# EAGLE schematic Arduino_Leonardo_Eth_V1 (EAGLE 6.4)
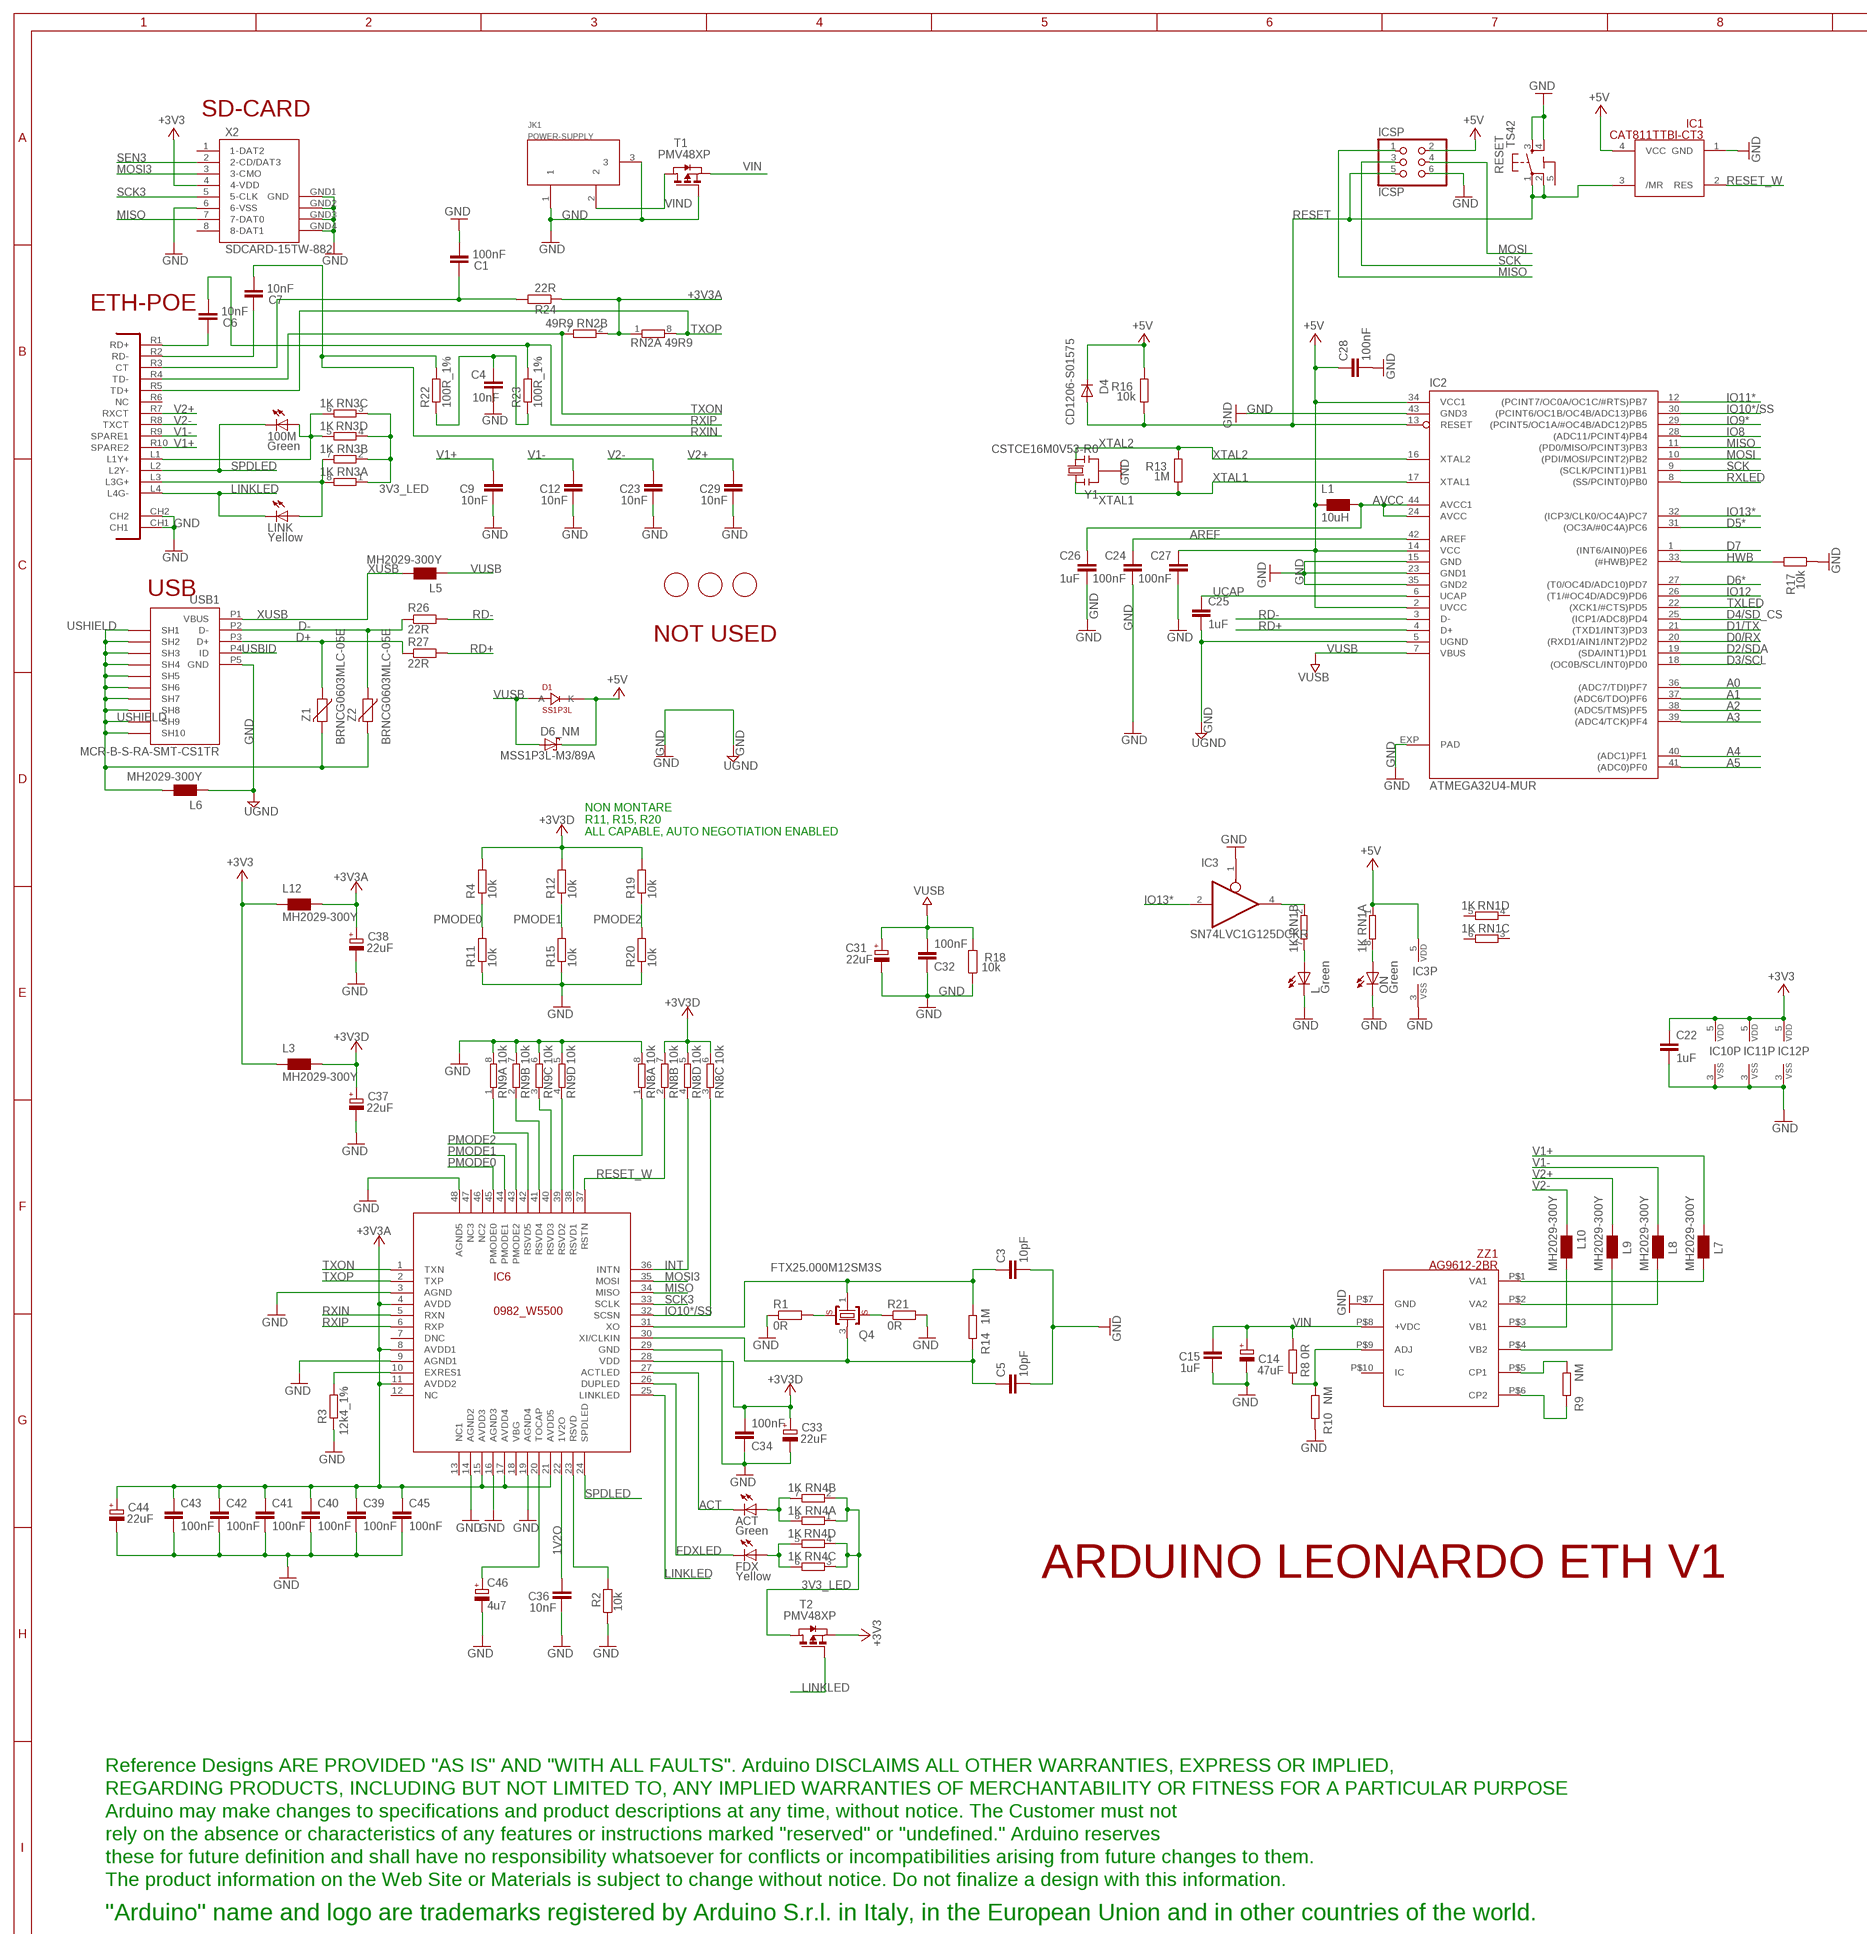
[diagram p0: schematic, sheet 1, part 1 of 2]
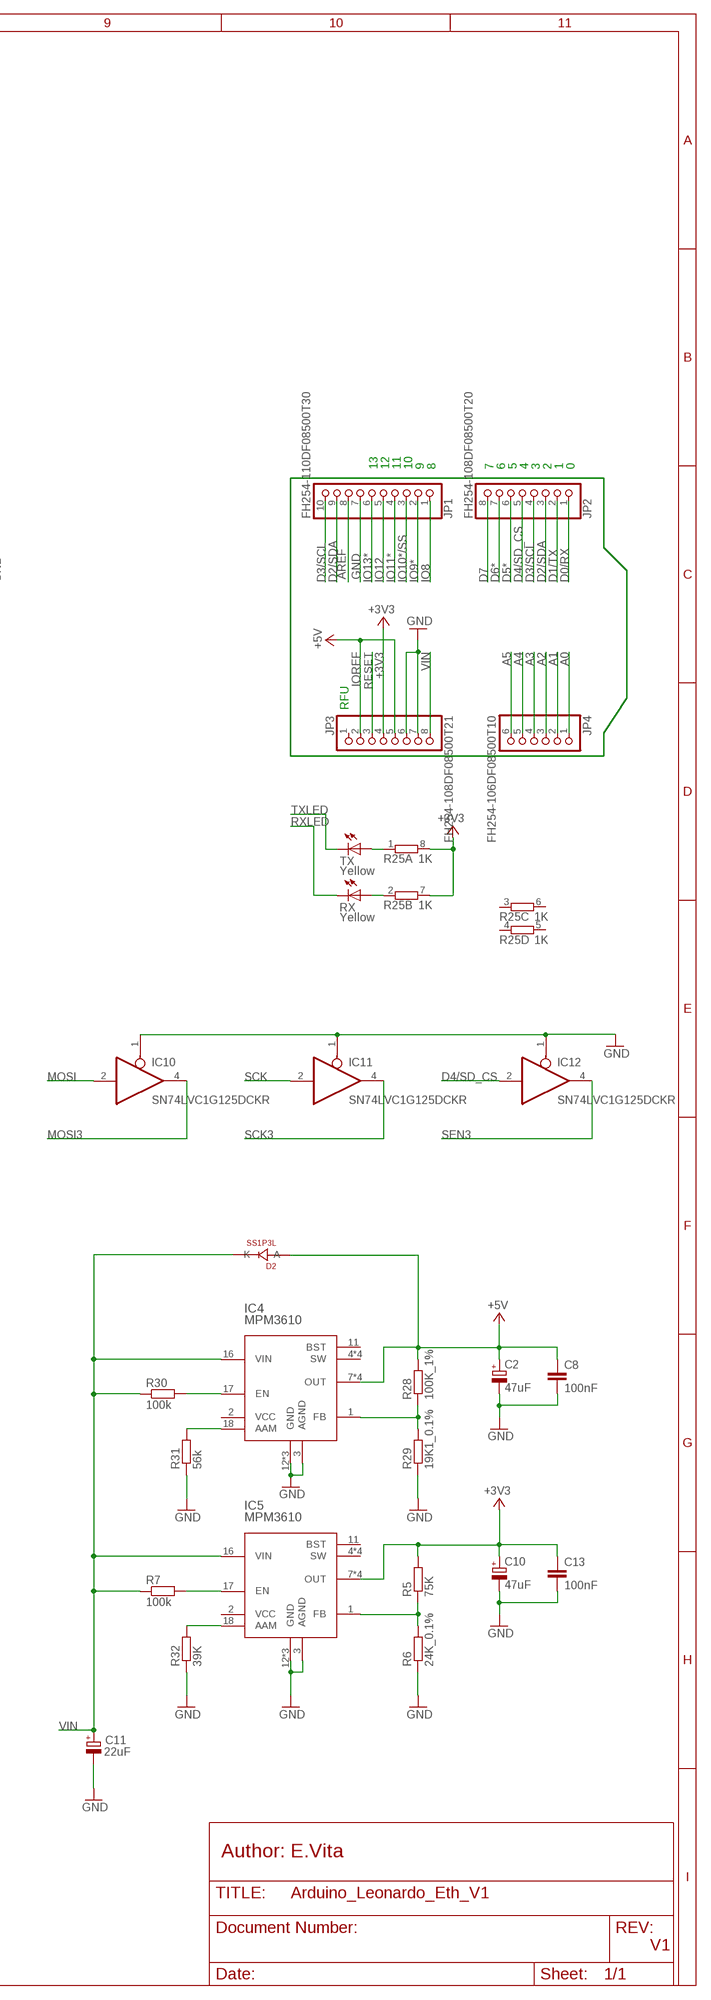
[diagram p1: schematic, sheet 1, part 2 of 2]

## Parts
100M  Green  0043_KPT-2012SGC  [CHIPLED_0805]
ACT  Green  0043_KPT-2012SGC  [CHIPLED_0805]
C1  100nF  0015_100NF_0603  [C0603-ROUND]
C2  47uF  0113_47UF  [PANASONIC_D]
C3  10pF  0245_0603C0G10PF50V  [C0603-ROUND]
C4  10nF  0142_10NF_0603  [C0603-ROUND]
C5  10pF  0245_0603C0G10PF50V  [C0603-ROUND]
C6  10nF  0142_10NF_0603  [C0603-ROUND]
C7  10nF  0142_10NF_0603  [C0603-ROUND]
C8  100nF  0015_100NF_0603  [C0603-ROUND]
C9  10nF  0461_10NF_0805  [C0805K]
C10  47uF  0113_47UF  [PANASONIC_D]
C11  22uF  0167_  [SMC_B]
C12  10nF  0461_10NF_0805  [C0805K]
C13  100nF  0015_100NF_0603  [C0603-ROUND]
C14  47uF  0113_47UF  [PANASONIC_D]
C15  1uF  0006_1UF_0603/GRM188R61E105KA12D  [C0603-ROUND]
C22  1uF  0006_1UF_0603/GRM188R61E105KA12D  [C0603-ROUND]
C23  10nF  0461_10NF_0805  [C0805K]
C24  100nF  0015_100NF_0603  [C0603-ROUND]
C25  1uF  0006_1UF_0603/GRM188R61E105KA12D  [C0603-ROUND]
C26  1uF  0006_1UF_0603/GRM188R61E105KA12D  [C0603-ROUND]
C27  100nF  0015_100NF_0603  [C0603-ROUND]
C28  100nF  0015_100NF_0603  [C0603-ROUND]
C29  10nF  0461_10NF_0805  [C0805K]
C31  22uF  0167_  [SMC_B]
C32  100nF  0015_100NF_0603  [C0603-ROUND]
C33  22uF  0167_  [SMC_B]
C34  100nF  0015_100NF_0603  [C0603-ROUND]
C36  10nF  0142_10NF_0603  [C0603-ROUND]
C37  22uF  0167_  [SMC_B]
C38  22uF  0167_  [SMC_B]
C39  100nF  0015_100NF_0603  [C0603-ROUND]
C40  100nF  0015_100NF_0603  [C0603-ROUND]
C41  100nF  0015_100NF_0603  [C0603-ROUND]
C42  100nF  0015_100NF_0603  [C0603-ROUND]
C43  100nF  0015_100NF_0603  [C0603-ROUND]
C44  22uF  0167_  [SMC_B]
C45  100nF  0015_100NF_0603  [C0603-ROUND]
C46  4u7  0474_TAJA475M016RNJ  [SMC_A]
D1  SS1P3L  0025_SS1P3L-M3/84A  [DO220AAL]
D2  SS1P3L  0025_SS1P3L-M3/84A  [DO220AAL]
D4  CD1206-S01575  0012_CD1206-S01575  [MINIMELF]
D6_NM  MSS1P3L-M3/89A  1653_MSS1P3L-M3/89A  [MICROSMP]
FDX  Yellow  0044_KPT-2012YC  [CHIPLED_0805]
IC1  CAT811TTBI-CT3  0035_CAT811TTBI-GT3  [SOT143]
IC2  ATMEGA32U4-MUR  0159_ATMEGA32U4-MUR  [QFN44ML7X7]
IC3  SN74LVC1G125DCKR  0040_SN74LVC1G125DCKR  [SC70-5]
IC4  MPM3610  2093_MPM3610GQV-P  [QFN-20]
IC5  MPM3610  2093_MPM3610GQV-P  [QFN-20]
IC6  0982_W5500  [TQFP48-7X7]
IC10  SN74LVC1G125DCKR  0040_SN74LVC1G125DCKR  [SC70-5]
IC11  SN74LVC1G125DCKR  0040_SN74LVC1G125DCKR  [SC70-5]
IC12  SN74LVC1G125DCKR  0040_SN74LVC1G125DCKR  [SC70-5]
ICSP  ICSP  0114_PH254-203DF118A00V  [2X03]
JK1  POWER-SUPPLY  0018_19746-POWER-SUPPLY  [POWERSUPPLY_DC-21MM]
JP1  FH254-110DF08500T30  1216_FH254-110DF08500T30  [1X10]
JP2  FH254-108DF08500T20  1218_FH254-108DF08500T20  [1X08]
JP3  FH254-108DF08500T21  1217_FH254-108DF08500T21  [1X08]
JP4  FH254-106DF08500T10  1215_FH254-106DF08500T10_STD  [1X06]
L  Green  0043_KPT-2012SGC  [CHIPLED_0805]
L1  10uH  0715_CV201210-100K  [0805]
L3  MH2029-300Y  0001_BLM21PG300SN1D_/_MH2029-300Y  [0805]
L5  MH2029-300Y  0001_BLM21PG300SN1D_/_MH2029-300Y  [0805]
L6  MH2029-300Y  0001_BLM21PG300SN1D_/_MH2029-300Y  [0805]
L7  MH2029-300Y  0001_BLM21PG300SN1D_/_MH2029-300Y  [0805]
L8  MH2029-300Y  0001_BLM21PG300SN1D_/_MH2029-300Y  [0805]
L9  MH2029-300Y  0001_BLM21PG300SN1D_/_MH2029-300Y  [0805]
L10  MH2029-300Y  0001_BLM21PG300SN1D_/_MH2029-300Y  [0805]
L12  MH2029-300Y  0001_BLM21PG300SN1D_/_MH2029-300Y  [0805]
LINK  Yellow  0044_KPT-2012YC  [CHIPLED_0805]
ON  Green  0043_KPT-2012SGC  [CHIPLED_0805]
Q4  FTX25.000M12SM3S  0846_FTX25.000M12SM3S  [CRYSTAL3.2X2.5]
R1  0R  0039_JUMP_0402  [R0402]
R2  10k  0028_CR0603JW103L  [R0603-ROUND]
R3  12k4_1%  0984_12K4_1%_0603  [R0603-ROUND]
R4  10k  0028_CR0603JW103L  [R0603-ROUND]
R5  75K  0376_CR0603FX7502_L  [R0603-ROUND]
R6  24K_0.1%  2338_  [R0603-ROUND]
R7  100k  0026_100K_0603  [R0603-ROUND]
R8  0R  0233_0R_0603  [R0603-ROUND]
R9  NM  0233_0R_0603  [R0603-ROUND]
R10  NM  0233_0R_0603  [R0603-ROUND]
R11  10k  0028_CR0603JW103L  [R0603-ROUND]
R12  10k  0028_CR0603JW103L  [R0603-ROUND]
R13  1M  0004_0603_1M  [R0603-ROUND]
R14  1M  0004_0603_1M  [R0603-ROUND]
R15  10k  0028_CR0603JW103L  [R0603-ROUND]
R16  10k  0028_CR0603JW103L  [R0603-ROUND]
R17  10k  0028_CR0603JW103L  [R0603-ROUND]
R18  10k  0028_CR0603JW103L  [R0603-ROUND]
R19  10k  0028_CR0603JW103L  [R0603-ROUND]
R20  10k  0028_CR0603JW103L  [R0603-ROUND]
R21  0R  0039_JUMP_0402  [R0402]
R22  100R_1%  0131_CR0603FX1000L  [R0603-ROUND]
R23  100R_1%  0131_CR0603FX1000L  [R0603-ROUND]
R24  22R  0247_22R_0603  [R0603-ROUND]
R25  1K  0005_064R_1K_/_CAY16-102J4LF  [CAY16]
R26  22R  0247_22R_0603  [R0603-ROUND]
R27  22R  0247_22R_0603  [R0603-ROUND]
R28  100K_1%  2022_CR0603FW104L  [R0603-ROUND]
R29  19K1_0.1%  2339_  [R0603-ROUND]
R30  100k  0026_100K_0603  [R0603-ROUND]
R31  56k  0411_56K_0603  [R0603-ROUND]
R32  39K  0756_  [R0603-ROUND]
RESET  TS42  0946_TS42031-160W-TR-7260  [TS42]
RN1  1K  0005_064R_1K_/_CAY16-102J4LF  [CAY16]
RN2  49R9  0036_CAY16-49R9F4L  [CAY16]
RN3  1K  0005_064R_1K_/_CAY16-102J4LF  [CAY16]
RN4  1K  0005_064R_1K_/_CAY16-102J4LF  [CAY16]
RN8  10k  0016_064R_10K_/_CAY16-103J4LF  [CAY16]
RN9  10k  0016_064R_10K_/_CAY16-103J4LF  [CAY16]
RX  Yellow  0044_KPT-2012YC  [CHIPLED_0805]
T1  PMV48XP  0297_PMV48XP  [SOT-23]
T2  PMV48XP  0297_PMV48XP  [SOT-23]
TX  Yellow  0044_KPT-2012YC  [CHIPLED_0805]
U$1  DISCLAIMER  [DISCLAIMER]
U$2  FIDUCIALMOUNT  [FIDUCIA-MOUNT]
U$4  FIDUCIALMOUNT  [FIDUCIA-MOUNT]
U$5  FIDUCIALMOUNT  [FIDUCIA-MOUNT]
UC1  RB1-125BHQ1A  0033_RB1-125BHQ1A  [POE-RJ45]
USB1  MCR-B-S-RA-SMT-CS1TR  0158_MCR-B-S-RA-SMT-CS1TR  [CON2_USB_MICRO_B_AT]
X2  SDCARD-15TW-882  0046_15TW-882  [SDCARD-15TW-8821]
Y1  CSTCE16M0V53-R0  0011_CSTCE16M0V53-R0  [RESONATOR]
Z1  BRNCG0603MLC-05E  0010_BRNCG0603MLC-05E  [CT/CN0603]
Z2  BRNCG0603MLC-05E  0010_BRNCG0603MLC-05E  [CT/CN0603]
ZZ1  AG9612-2BR  0343_AG9612-2BR  [AG9000]

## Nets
1V2O: C36.2 IC6.22(1V2O)
3V3_LED [power]: RN3.1 RN3.2 RN3.3 RN3.4 RN4.1 RN4.2 RN4.3 RN4.4 T2.1(D)
+3V3 [power]: C10.+ C13.1 C22.1 IC5.7(OUT) IC5.8(OUT) IC5.9(OUT) IC5.20(OUT) IC10.5(VDD) IC11.5(VDD) IC12.5(VDD) JP3.4 L3.1 L12.1 R5.2 R25.7 R25.8 T2.2(S) X2.4(4-VDD)
+3V3A [power]: C38.+ C39.1 C40.1 C41.1 C42.1 C43.1 C44.+ C45.1 IC6.4(AVDD) IC6.8(AVDD1) IC6.11(AVDD2) IC6.15(AVDD3) IC6.17(AVDD4) IC6.21(AVDD5) L12.2 R24.1 RN2.1 RN2.2
+3V3D: C33.+ C34.2 C37.+ IC6.28(VDD) L3.2 R4.2 R12.2 R19.2 RN8.5 RN8.6 RN8.7
+5V [power]: C2.+ C8.1 C27.2 C28.1 D1.P$1(K) D2.P$2(A) D4.C D6_NM.K(C) IC1.4(VCC) IC2.2(UVCC) IC2.14(VCC) IC2.34(VCC1) IC3.5(VDD) IC4.7(OUT) IC4.8(OUT) IC4.9(OUT) IC4.20(OUT) ICSP.2 JP3.2 JP3.5 L1.1 R16.2 R28.2 RN1.1
A0: IC2.36((ADC7/TDI)PF7) JP4.1
A1: IC2.37((ADC6/TDO)PF6) JP4.2
A2: IC2.38((ADC5/TMS)PF5) JP4.3
A3: IC2.39((ADC4/TCK)PF4) JP4.4
A4: IC2.40((ADC1)PF1) JP4.5
A5: IC2.41((ADC0)PF0) JP4.6
ACT: ACT.C IC6.27(ACTLED)
AREF: C24.2 IC2.42(AREF) JP1.8
AVCC: C26.1 IC2.24(AVCC) IC2.44(AVCC1) L1.2
D0/RX: IC2.20((RXD1/AIN1/INT2)PD2) JP2.1
D1/TX: IC2.21((TXD1/INT3)PD3) JP2.2
D2/SDA: IC2.19((SDA/INT1)PD1) JP1.9 JP2.3
D3/SCL: IC2.18((OC0B/SCL/INT0)PD0) JP1.10 JP2.4
D4/SD_CS: IC2.25((ICP1/ADC8)PD4) IC12.2(I) JP2.5
D5*: IC2.31((OC3A/#0C4A)PC6) JP2.6
D6*: IC2.27((T0/OC4D/ADC10)PD7) JP2.7
D7: IC2.1((INT6/AIN0)PE6) JP2.8
D+: R27.1 USB1.P3(D+) Z1.1
D-: R26.1 USB1.P2(D-) Z2.1
FDXLED: FDX.C IC6.26(DUPLED)
GND [power]: C1.1 C2.- C3.2 C4.1 C5.2 C8.2 C9.1 C10.- C11.- C12.1 C13.2 C14.- C15.1 C22.2 C23.1 C24.1 C25.2 C26.2 C27.1 C28.2 C29.1 C31.- C32.1 C33.- C34.1 C36.1 C37.- C38.- C39.2 C40.2 C41.2 C42.2 C43.2 C44.- C45.2 C46.- IC1.1(GND) IC2.5(UGND) IC2.15(GND) IC2.23(GND1) IC2.35(GND2) IC2.43(GND3) IC2.EXP(PAD) IC3.1(OE) IC3.3(VSS) IC4.3(AGND) IC4.12(GND) IC4.13(GND) IC4.14(GND) IC5.3(AGND) IC5.12(GND) IC5.13(GND) IC5.14(GND) IC6.3(AGND) IC6.9(AGND1) IC6.14(AGND2) IC6.16(AGND3) IC6.19(AGND4) IC6.29(GND) IC6.48(AGND5) IC10.1(OE) IC10.3(VSS) IC11.1(OE) IC11.3(VSS) IC12.1(OE) IC12.3(VSS) ICSP.6 JK1.1 JK1.3 JP1.7 JP3.6 JP3.7 L6.1 L.C ON.C R1.1 R2.1 R3.1 R6.1 R10.2 R11.1 R15.1 R17.1 R18.1 R20.1 R21.2 R29.1 R31.1 R32.1 RESET.3 RESET.4 RN8.8 RN9.5 RN9.6 RN9.7 RN9.8 T1.3(G) UC1.CH1 UC1.CH2 USB1.P5(GND) X2.6(6-VSS) X2.GND1(GND) X2.GND2(GND1) X2.GND3(GND2) X2.GND4(GND3) Y1.2 ZZ1.P$7(GND) ; supply symbol labelled UGND
HWB: IC2.33((#HWB)PE2) R17.2
INT: IC6.36(INTN) RN8.4
IO8: IC2.28((ADC11/PCINT4)PB4) JP1.1
IO9*: IC2.29((PCINT5/OC1A/#OC4B/ADC12)PB5) JP1.2
IO10*/SS: IC2.30((PCINT6/OC1B/OC4B/ADC13)PB6) IC6.32(SCSN) JP1.3 RN8.3
IO11*: IC2.12((PCINT7/OC0A/OC1C/#RTS)PB7) JP1.4
IO12: IC2.26((T1/#OC4D/ADC9)PD6) JP1.5
IO13*: IC2.32((ICP3/CLK0/OC4A)PC7) IC3.2(I) JP1.6
LINKLED: IC6.25(LINKLED) LINK.C T2.3(G) UC1.L4(L4G-)
MISO: IC2.11((PD0/MISO/PCINT3)PB3) IC6.34(MISO) ICSP.1 X2.7(7-DAT0)
MOSI: IC2.10((PDI/MOSI/PCINT2)PB2) IC10.2(I) ICSP.4
MOSI3: IC6.35(MOSI) IC10.4(O) X2.3(3-CMO)
N$1: IC3.4(O) RN1.2
N$2: LINK.A RN3.7 RN3.8 UC1.L3(L3G+)
N$3: 100M.A RN3.5 RN3.6 UC1.L1(L1Y+)
N$5: L.A RN1.7
N$6: R25.1 TX.A
N$7: R25.2 RX.A
N$8: ON.A RN1.8
N$9: ACT.A RN4.7 RN4.8
N$10 [power]: C1.2 R24.2 UC1.R3(CT)
N$12: C3.1 IC6.31(XO) Q4.1 R14.1
N$13 [ETH]: L10.2 ZZ1.P$3(VB1)
N$14 [ETH]: L9.2 ZZ1.P$4(VB2)
N$15 [ETH]: L8.2 ZZ1.P$2(VA2)
N$16 [ETH]: L7.2 ZZ1.P$1(VA1)
N$17: Q4.2 R1.2
N$18: Q4.4 R21.1
N$19: C6.2 UC1.R1(RD+)
N$20: IC6.39(RSVD2) RN9.4
N$21: C4.2 R22.1 R23.1
N$22: C7.2 UC1.R2(RD-)
N$24: IC6.23(RSVD) R2.2
N$25: IC5.1(FB) R5.1 R6.2
N$26: IC4.1(FB) R28.1 R29.2
N$27: IC5.17(EN) R7.2
N$28: IC4.17(EN) R30.2
N$29: IC4.18(AAM) R31.2
N$30: FDX.A RN4.5 RN4.6
N$31: IC6.40(RSVD3) RN9.3
N$32: R9.1 ZZ1.P$5(CP1)
N$33: R9.2 ZZ1.P$6(CP2)
N$34: R8.2 R10.1 ZZ1.P$9(ADJ)
N$35: IC6.41(RSVD4) RN9.2
N$36: IC5.18(AAM) R32.2
N$37: IC6.42(RSVD5) RN9.1
N$38: C46.+ IC6.20(TOCAP)
N$39: IC6.38(RSVD1) RN8.1
N$40: IC6.10(EXRES1) R3.2
OSC2E1: C5.1 IC6.30(XI/CLKIN) Q4.3 R14.2
PMODE0: IC6.45(PMODE0) R4.1 R11.2
PMODE1: IC6.44(PMODE1) R12.1 R15.2
PMODE2: IC6.43(PMODE2) R19.1 R20.2
RD+: IC2.4(D+) R27.2
RD-: IC2.3(D-) R26.2
RESET: D4.A IC1.3(/MR) IC2.13(RESET) ICSP.5 JP3.3 R16.1 RESET.1 RESET.2
RESET_W: IC1.2(RES) IC6.37(RSTN) RN8.2
RXIN: C7.1 IC6.5(RXN) R22.2
RXIP: C6.1 IC6.6(RXP) R23.2
RXLED: IC2.8((SS/PCINT0)PB0) RX.C
SCK: IC2.9((SCLK/PCINT1)PB1) IC11.2(I) ICSP.3
SCK3: IC6.33(SCLK) IC11.4(O) X2.5(5-CLK)
SEN3: IC12.4(O) X2.2(2-CD/DAT3)
SPDLED: 100M.C IC6.24(SPDLED) UC1.L2(L2Y-)
TXLED: IC2.22((XCK1/#CTS)PD5) TX.C
TXON: IC6.1(TXN) RN2.7 UC1.R4(TD-)
TXOP: IC6.2(TXP) RN2.8 UC1.R5(TD+)
UCAP: C25.1 IC2.6(UCAP)
USBID: USB1.P4(ID)
USHIELD [gnd]: L6.2 USB1.P$1(SH7) USB1.P$2(SH8) USB1.P$3(SH9) USB1.P$4(SH10) USB1.P$5(SH7) USB1.P$6(SH8) USB1.P$7(SH9) USB1.P$8(SH10) USB1.S1(SH1) USB1.S2(SH2) USB1.S3(SH3) USB1.S4(SH4) USB1.S5(SH5) USB1.S6(SH6) Z1.2 Z2.2
V1+ [ETH]: C9.2 L7.1 UC1.R10(SPARE2)
V1- [ETH]: C12.2 L8.1 UC1.R9(SPARE1)
V2+ [ETH]: C29.2 L9.1 UC1.R7(RXCT)
V2- [ETH]: C23.2 L10.1 UC1.R8(TXCT)
VIN [gnd]: C11.+ C14.+ C15.2 D2.P$1(K) IC4.16(VIN) IC5.16(VIN) JP3.8 R7.1 R8.1 R30.1 T1.2(S) ZZ1.P$8(+VDC)
VIND [gnd]: JK1.2 T1.1(D)
VUSB: C31.+ C32.2 D1.P$2(A) D6_NM.A IC2.7(VBUS) L5.1 R18.2
XTAL1: IC2.17(XTAL1) R13.1 Y1.1
XTAL2: IC2.16(XTAL2) R13.2 Y1.3
XUSB [usbvcc]: L5.2 USB1.P1(VBUS)
Unconnected: IC4.2(VCC) IC4.4(SW) IC4.5(SW) IC4.6(SW) IC4.11(BST) IC4.19(SW) IC5.2(VCC) IC5.4(SW) IC5.5(SW) IC5.6(SW) IC5.11(BST) IC5.19(SW) IC6.7(DNC) IC6.13(NC1) IC6.18(VBG) IC6.46(NC2) IC6.47(NC3) JP3.1 R25.3 R25.4 R25.5 R25.6 RN1.3 RN1.4 RN1.5 RN1.6 RN2.3 RN2.4 RN2.5 RN2.6 UC1.R6(NC) X2.1(1-DAT2) X2.8(8-DAT1) ZZ1.P$10(IC)

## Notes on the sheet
- SD-CARD
- ETH-POE
- 13 | 12 | 11 | 10 | 9 | 8 | 7 | 6 | 5 | 4 | 3 | 2 | 1 | 0
- USB
- NOT USED
- IOREF
- RFU
- NON MONTARE
  R11, R15, R20
  ALL CAPABLE, AUTO NEGOTIATION ENABLED
- ARDUINO LEONARDO ETH V1
- Author: E.Vita
- V1

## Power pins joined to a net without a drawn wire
5-GND: RESET.5(5-GND)
NC: IC6.12(NC)

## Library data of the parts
100M ACT L ON = Opto:0043_KPT-2012SGC: LED GREEN - SMD-0805; MONTHLY_USAGE: _____; PART_NUMBER: KPT-2012SGC; PRICE: _____; SUPPLIER: _____; TYPE: Opto
C1 C8 C13 C24 C27 C28 C32 C34 C39-C43 C45 = Condensatori:0015_100NF_0603: 100nF 0603 50V; CASE: 0603; MONTHLY_USAGE: _____; PART_NUMBER: cl10b104kbnc; PRICE: _____; SUPPLIER: _____; TYPE: Condensatori
C2 C10 C14 = Condensatori:0113_47UF: 47uF; MONTHLY_USAGE: _____; PART_NUMBER: 47uF; PRICE: _____; SUPPLIER: _____; TYPE: Condensatori
C3 C5 = Condensatori:0245_0603C0G10PF50V: 10pF 0603; CASE: 0603; MONTHLY_USAGE: _____; PART_NUMBER: 0603C0G10PF50V; PRICE: _____; SUPPLIER: _____; TYPE: Condensatori
C4 C6 C7 C36 = Condensatori:0142_10NF_0603: 10nF 0603; CASE: 0603; MONTHLY_USAGE: _____; PART_NUMBER: 10nF_0603; PRICE: _____; SUPPLIER: _____; TYPE: Condensatori
C9 C12 C23 C29 = Condensatori:0461_10NF_0805: 10nF 0805; CASE: 0805; MONTHLY_USAGE: _____; PART_NUMBER: 10nF_0805; PRICE: _____; SUPPLIER: _____; TYPE: Condensatori
C11 C31 C33 C37 C38 C44 = Condensatori:0167_: 22uF 25V; MONTHLY_USAGE: _____; PRICE: _____; SUPPLIER: _____; TYPE: Condensatori
C15 C22 C25 C26 = Condensatori:0006_1UF_0603/GRM188R61E105KA12D: 1uF 0603; CASE: 0603; MONTHLY_USAGE: _____; PART_NUMBER: 1uF_0603/GRM188R61E105KA12D; PRICE: _____; SUPPLIER: _____; TYPE: Condensatori
C46 = Condensatori:0474_TAJA475M016RNJ: 4u7 tantalio Case A - testa gialla -Tantalio; CASE: CaseA_(1206); MONTHLY_USAGE: _____; PART_NUMBER: TAJA475M016RNJ; PRICE: _____; SUPPLIER: _____; TYPE: Condensatori
D1 D2 = Diodi:0025_SS1P3L-M3/84A: 1A 30V Schottky Barrier Rectifiers -SS1P3L-M3/84A; CASE: SMP; MONTHLY_USAGE: _____; PART_NUMBER: SS1P3L-M3/84A; PRICE: _____; SUPPLIER: _____; TYPE: Diodi
D4 = Diodi:0012_CD1206-S01575: small-signal high-speed Switching Diodes CD1206; CASE: 1206; MONTHLY_USAGE: _____; PART_NUMBER: CD1206-S01575; PRICE: _____; SUPPLIER: _____; TYPE: Diodi
D6_NM = Diodi:1653_MSS1P3L-M3/89A: Surface Mount Schottky Barrier Rectifiers - Case microSMP
FDX LINK RX TX = Opto:0044_KPT-2012YC: LED YELLOW - SMD - 0805; MONTHLY_USAGE: _____; PART_NUMBER: KPT-2012YC; PRICE: _____; SUPPLIER: _____; TYPE: Opto
IC1 = Circuito Integrato:0035_CAT811TTBI-GT3: 4-Pin Microprocessor Power Supply Supervisors- Reset Controller CAT811TTBI-GT3; CASE: SOT143-4; MONTHLY_USAGE: _____; PART_NUMBER: CAT811TTBI-GT3; PRICE: _____; SUPPLIER: _____; TYPE: Circuito_Integrato; VALUE: CAT811TTBI-GT3
IC2 = IntegratedCircuits:0159_ATMEGA32U4-MUR: 8-bit Microcontroller with 32K Bytes of ISP Flash and USB Controller ATMEGA32U4-MUR; CASE: QFN44_7x7; PART_NUMBER: ATMEGA32U4-MUR; TYPE: Circuito_Integrato
IC3 IC10-IC12 = Circuito Integrato:0040_SN74LVC1G125DCKR: Single bus buffer with 3-state output; CASE: SC70; MONTHLY_USAGE: _____; PART_NUMBER: SN74LVC1G125DCKR; PRICE: _____; SUPPLIER: _____; TYPE: Circuito_Integrato; VALUE: 74LVC1G125DCKR
IC4 IC5 = IntegratedCircuits:2093_MPM3610GQV-P: MPM3610 Step Down Regulator; CASE: QFN-20; PART_NUMBER: MPM3610GQV-P; TYPE: Circuito_Integrato
IC6 = Circuito Integrato:0982_W5500: The W5500 chip is a Hardwired TCP/IP embedded Ethernet controller that enables easier internet connection for embedded systems using SPI (Serial Peripheral Interface). Case TQFP48; PART_NUMBER: W5500
ICSP = Connettori:0114_PH254-203DF118A00V: 3x2 M V h 8,5 mm p2,54; MONTHLY_USAGE: _____; PART_NUMBER: PH254-203DF118A00V; PRICE: _____; SUPPLIER: _____; TYPE: Connettori
JK1 = Connettori:0018_19746-POWER-SUPPLY: JACK; MONTHLY_USAGE: _____; PART_NUMBER: 19746; PRICE: _____; SUPPLIER: _____; TYPE: Connettori
JP1 = Connettori:1216_FH254-110DF08500T30: Female Connector strip for Arduino bases - 10x1 F V h 8,5 p2,54 serigrafato STRISCIA VUOTA; MONTHLY_USAGE: _____; PART_NUMBER: FH254-110DF08500T30; PRICE: _____; SUPPLIER: _____; TYPE: Connettori
JP2 = Connettori:1218_FH254-108DF08500T20: Female Connector strip for Arduino bases - 8x1 F V h 8,5 p2,54 serigrafato DIGITAL; MONTHLY_USAGE: _____; PART_NUMBER: FH254-108DF08500T20; PRICE: _____; SUPPLIER: _____; TYPE: Connettori
JP3 = Connettori:1217_FH254-108DF08500T21: Female Connector strip for Arduino bases - 8x1 F V h 8,5 p2,54 serigrafato POWER; MONTHLY_USAGE: _____; PART_NUMBER: FH254-108DF08500T21; PRICE: _____; SUPPLIER: _____; TYPE: Connettori
JP4 = Connettori:1215_FH254-106DF08500T10: Female Connector strip for Arduino Boards - 6x1 F V h 8,5 p2,54 serigrafato ANALOG IN; MONTHLY_USAGE: 86722.85; PART_NUMBER: FH254-106DF08500T10; PRICE: _0.03; SUPPLIER: CBC_elettronica__s.r.l.; TYPE: Connettori
L1 = Induttanze:0715_CV201210-100K: 10uH 0805; CASE: 0805; MONTHLY_USAGE: _____; PART_NUMBER: CV201210-100K; PRICE: _____; SUPPLIER: _____; TYPE: Induttanze
L3 L5-L10 L12 = Protezione:0001_BLM21PG300SN1D_/_MH2029-300Y: BLM21; MONTHLY_USAGE: _____; PART_NUMBER: BLM21PG300SN1D_/_MH2029-300Y; PRICE: _____; SUPPLIER: _____; TYPE: Protezione
Q4 = Cristalli:0846_FTX25.000M12SM3S: 25Mhz - K7 12pF - SMD; MONTHLY_USAGE: _____; PART_NUMBER: FTX25.000M12SM3S; PRICE: _____; SUPPLIER: _____; TYPE: Cristalli
R1 R21 = Resistenze:0039_JUMP_0402: 0R 0402; CASE: 0402; MONTHLY_USAGE: _____; PART_NUMBER: JUMP_0402; PRICE: _____; SUPPLIER: _____; TYPE: Resistenze
R2 R4 R11 R12 R15-R20 = Resistenze:0028_CR0603JW103L: 10K 0603; CASE: 0603; MONTHLY_USAGE: _____; PART_NUMBER: CR0603JW103L; PRICE: _____; SUPPLIER: _____; TYPE: Resistenze
R3 = Resistenze:0984_12K4_1%_0603: 12K4 1% 0603; CASE: 0603; MONTHLY_USAGE: _____; PART_NUMBER: 12K4_1%_0603; PRICE: _____; SUPPLIER: _____; TYPE: Resistenze
R5 = Resistenze:0376_CR0603FX7502_L: 75K 0603; CASE: 0603; MONTHLY_USAGE: _____; PART_NUMBER: CR0603FX7502_L; PRICE: _____; SUPPLIER: _____; TYPE: Resistenze
R6 = Resistenze:2338_: 24K 0,1% 0603; CASE: 0603; MONTHLY_USAGE: _____; PRICE: _____; SUPPLIER: _____; TYPE: Resistenze; VALUE: 24K_0,1%
R7 R30 = Resistenze:0026_100K_0603: 100K 0603; CASE: 0603; MONTHLY_USAGE: _____; PART_NUMBER: 100K_0603; PRICE: _____; SUPPLIER: _____; TYPE: Resistenze
R8 = Resistenze:0233_0R_0603: 0R 0603; CASE: 0603; MONTHLY_USAGE: _____; PART_NUMBER: 0R_0603; PRICE: _____; SUPPLIER: _____; TYPE: Resistenze
R9 R10 = Resistenze:0233_0R_0603: 0R 0603; CASE: 0603; MONTHLY_USAGE: _____; PART_NUMBER: 0R_0603; PRICE: _____; SUPPLIER: _____; TYPE: Resistenze; VALUE: 0R
R13 R14 = Resistenze:0004_0603_1M: 1M 0603; CASE: 0603; MONTHLY_USAGE: _____; PART_NUMBER: 0603_1M; PRICE: _____; SUPPLIER: _____; TYPE: Resistenze
R22 R23 = Resistenze:0131_CR0603FX1000L: Resistenza SMD 100R 0603 1%; CASE: 0603; PART_NUMBER: CR0603FX1000L; TYPE: Resistenze
R24 R26 R27 = Resistenze:0247_22R_0603: 22R 0603; CASE: 0603; MONTHLY_USAGE: _____; PART_NUMBER: 22R_0603; PRICE: _____; SUPPLIER: _____; TYPE: Resistenze
R25 RN1 RN3 RN4 = Resistenze:0005_064R_1K_/_CAY16-102J4LF: 1K 064R; CASE: SMD_3,2x1,6; MONTHLY_USAGE: _____; PART_NUMBER: 064R_1K_/_CAY16-102J4LF; PRICE: _____; SUPPLIER: _____; TYPE: Resistenze
R28 = Resistenze:2022_CR0603FW104L: 0603 Resistor 100K 1%; PART_NUMBER: CR0603FW104L
R29 = Resistenze:2339_: 19K1 0,1% 0603; CASE: 0603; MONTHLY_USAGE: _____; PRICE: _____; SUPPLIER: _____; TYPE: Resistenze; VALUE: 19K1_0,1%
R31 = Resistenze:0411_56K_0603: 56K 0603; CASE: 0603; MONTHLY_USAGE: _____; PART_NUMBER: 56K_0603; PRICE: _____; SUPPLIER: _____; TYPE: Resistenze
R32 = Resistenze:0756_: 39K 0603; CASE: 0603; MONTHLY_USAGE: _____; PRICE: _____; SUPPLIER: _____; TYPE: Resistenze
RESET = Switches:0946_TS42031-160W-TR-7260: Pushbutton 6x6 Smd - White; MONTHLY_USAGE: _____; PART_NUMBER: IT-1157AHNP-160G-G_GTR; PRICE: _____; SUPPLIER: _____; TYPE: Switches
RN2 = Resistenze:0036_CAY16-49R9F4L: 49R9; CASE: SMD_3,2x1,6; MONTHLY_USAGE: _____; PART_NUMBER: CAY16-49R9F4L; PRICE: _____; SUPPLIER: _____; TYPE: Resistenze
RN8 RN9 = Resistenze:0016_064R_10K_/_CAY16-103J4LF: 10K 064 R; CASE: SMD_3,2x1,6; MONTHLY_USAGE: _____; PART_NUMBER: 064R_10K_/_CAY16-103J4LF; PRICE: _____; SUPPLIER: _____; TYPE: Resistenze
T1 T2 = Transistors:0297_PMV48XP: 20 V, 3.5 A P-channel Trench MOSFET - PMV48XP; CASE: SOT23; MONTHLY_USAGE: _____; PART_NUMBER: PMV48XP; PRICE: _____; SUPPLIER: _____; TYPE: Transistor
U$1 = Misc:DISCLAIMER
U$2 U$4 U$5 = SmartPrj:FIDUCIALMOUNT
UC1 = Connettori:0033_RB1-125BHQ1A: RB1-125BHQ1A; MONTHLY_USAGE: _____; PART_NUMBER: RB1-125BHQ1A; PRICE: _____; SUPPLIER: _____; TYPE: Connettori
USB1 = Connettori:0158_MCR-B-S-RA-SMT-CS1TR: Usb Micro F/90 Smd Tipo B; MONTHLY_USAGE: _____; PART_NUMBER: MCR-B-S-RA-SMT-CS1TR; PRICE: _____; SUPPLIER: _____; TYPE: Connettori
X2 = Connettori:0046_15TW-882: SD CARD MICRO SMD-15TW-15882; MONTHLY_USAGE: _____; PART_NUMBER: 15TW-882 REEL; PRICE: _____; SUPPLIER: _____; TYPE: Connettori
Y1 = Cristalli:0011_CSTCE16M0V53-R0: 16Mhz - SMD; MONTHLY_USAGE: _____; PART_NUMBER: CSTCE16M0V53-R0; PRICE: _____; SUPPLIER: _____; TYPE: Cristalli
Z1 Z2 = Protezione:0010_BRNCG0603MLC-05E: CG0603MLC-05E; MONTHLY_USAGE: _____; PART_NUMBER: BRNCG0603MLC-05E; PRICE: _____; SUPPLIER: _____; TYPE: Protezione
ZZ1 = Moduli:0343_AG9612-2BR: Poe module AG9612-2BR, 12V, isolato; MONTHLY_USAGE: _____; PART_NUMBER: AG9612-2BR; PRICE: _____; SUPPLIER: _____; TYPE: Moduli

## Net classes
0 default: width 0.254 mm, drill 0.508 mm, clearance 0.102 mm
1 power: width 0.254 mm, drill 0.508 mm, clearance 0.203 mm
2 gnd: width 0.254 mm, drill 0.508 mm, clearance 0.254 mm
3 usbvcc: width 0.254 mm, drill 0.508 mm, clearance 0.254 mm
4 aref: width 0.254 mm, drill 0.508 mm, clearance 0.203 mm
5 ETH: width 0.305 mm, drill 0.508 mm, clearance 0.762 mm to class 0, clearance 0.762 mm to class 1, clearance 0.762 mm to class 2, clearance 0.762 mm to class 3, clearance 0.762 mm to class 4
